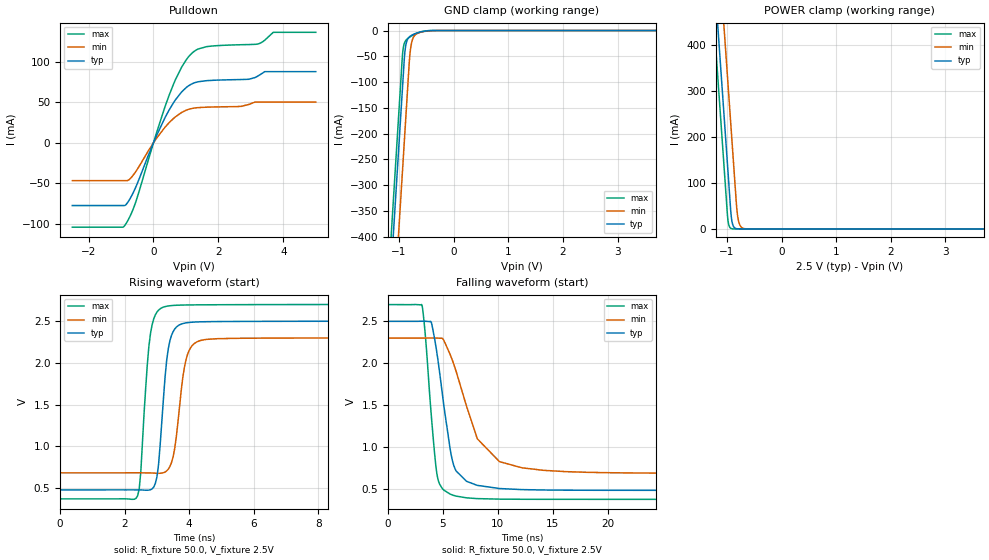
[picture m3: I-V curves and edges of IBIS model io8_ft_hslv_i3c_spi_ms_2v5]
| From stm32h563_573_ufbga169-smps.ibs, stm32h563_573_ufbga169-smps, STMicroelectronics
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[Model]   io8_ft_hslv_i3c_spi_ms_2v5
Model_type I/O_open_drain
Polarity   Non-Inverting
Enable   Active-Low
| CAP_THRESHOLD on pad IOFT is "UDTCAPC" :
| Rising=20.0% of vddiom   Falling=80.0% of vddiom
| C_comp min and max val. don't necessarily correlate with the min and max pvt
| but are the smallest and greatest pad capacitance found.
| var   typ   min   max
C_comp   3.87733pF  3.87281pF  3.96694pF
|C_comp_pulldown   3.87733pF  3.87281pF  3.96694pF
Vinl = 1.15V
Vinh = 1.35V
Vmeas = 1.25V   | Reference voltage for timing measurements
Cref  = 50.0pF   | Timing specification test load capacitance value
Rref  = 1.0MOhm   | Timing specification test load resistance value
Vref  = 1.375V   | Timing specification test load voltage
[Model Spec]
| TIME_THRESHOLD on pin ZII2CV11 is "CMOS" :
| Rising=40.0% of vdd   Falling=60.0% of vdd
Vinl 989.80000mV 917.80000mV 1.06580V
Vinh 1.40320V 1.29620V 1.49120V
| variable   typ   min   max
[Temperature Range] 25.0 125.0 -40.0
| variable   typ   min   max
[Voltage Range] 2.5V 2.3V 2.7V
| variable   typ   min   max
[POWER Clamp Reference] 2.5V 2.3V 2.7V
| variable   typ   min   max
[GND Clamp Reference] 0V 0V 0V
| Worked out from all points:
|   slope of the pulldown table from 0 to 0.375 V, typ, clamps not added: 11.5 ohm
|   GND clamp passes 1 mA (typ) near -0.52 V on its own axis
|   POWER clamp passes 1 mA (typ) near -0.84 V on its own axis
|   rising waveform, R_fixture 50.0, V_fixture 2.5V: 20-80 % time 254ps typ, 305ps min, 242ps max; typ from 0.481 V to 2.5 V
|   falling waveform, R_fixture 50.0, V_fixture 2.5V: 20-80 % time 1.3ns typ, 2.77ns min, 844ps max; typ from 2.5 V to 0.481 V
[POWER Clamp]
-2.5V     2.708A     2.899A     2.597A
-1.23V    548.8mA    740.2mA    437.5mA
-1.16V    429.8mA    621.2mA    318.5mA
-1.12V    361.8mA    553.2mA    250.5mA
-1.03V    208.8mA    400.2mA    97.53mA
-980mV    123.8mA    315.2mA    17.95mA
-920mV    26.3mA     213.2mA    906uA
-880mV    5.543mA    145.2mA    123.7uA
-810mV    363.5uA    33.6mA     3.797uA
-770mV    76.62uA    10.47mA    518.8nA
-700mV    5.026uA    1.361mA    16.11nA
5V        0A         0A         0A
[GND Clamp]
-2.5V     -2.77A     -2.931A    -2.704A
-1.21V    -576.8mA   -738.1mA   -511.3mA
-950mV    -134.8mA   -296.1mA   -69.34mA
-920mV    -83.82mA   -245.1mA   -32.48mA
-900mV    -50.56mA   -211.1mA   -24.02mA
-880mV    -31.31mA   -177.1mA   -19.85mA
-850mV    -18.7mA    -126.1mA   -16.34mA
-800mV    -11.46mA   -46.18mA   -12.45mA
-750mV    -8.203mA   -16.63mA   -9.325mA
-650mV    -4.063mA   -4.987mA   -4.427mA
-360mV    -35.05uA   -165.1uA   -9.564uA
5V        7.96nA     1.281uA    294pA
| variable   typ   min   max
[Pullup Reference] 2.5V 2.3V 2.7V
| variable   typ   min   max
[Pulldown Reference] 0V 0V 0V
[Pulldown]
-2.5V     -77.63mA   -46.85mA   -104.3mA
-870mV    -77.24mA   -46.85mA   -101.4mA
-550mV    -55.3mA    -35.88mA   -73.72mA
90mV      8.401mA    5.299mA    11.79mA
610mV     49.03mA    29.76mA    71.69mA
870mV     62.92mA    37.48mA    93.62mA
1.23V     73.63mA    42.72mA    112.2mA
1.64V     76.78mA    44.01mA    118.8mA
2.7V      78.15mA    44.99mA    121.2mA
3.22V     82.58mA    50.35mA    122.2mA
3.69V     87.93mA    50.35mA    136.5mA
5V        87.93mA    50.35mA    136.5mA
[Ramp]
dV/dt_r 1.21162V/249.69935ps 969.22666mV/302.34194ps 1.39626V/238.71411ps
dV/dt_f 1.21165V/1.30237ns 969.26055mV/2.47948ns 1.39628V/843.263ps
R_load = 50.0
| Removed startup time: 0s 0s 0s  .
| Removed end time: 34.4ns.
[Rising Waveform]
R_fixture   = 50.0
V_fixture   = 2.5V
V_fixture_min = 2.3V
V_fixture_max = 2.7V
0s        480.6mV    684.6mV    372.9mV
2.4ns     480.4mV    684.7mV    409.7mV
2.5ns     480mV      684.6mV    696.6mV
2.8ns     481.7mV    683.1mV    2.352V
3.05ns    783.7mV    678.8mV    2.632V
3.35ns    2.167V     727.8mV    2.682V
3.55ns    2.406V     973.3mV    2.69V
3.9ns     2.48V      2.037V     2.694V
4.5ns     2.494V     2.28V      2.696V
34.4ns    2.5V       2.3V       2.7V
| Removed startup time: 0s 0s 0s  .
| Removed end time: 99.4ns.
[Falling Waveform]
R_fixture   = 50.0
V_fixture   = 2.5V
V_fixture_min = 2.3V
V_fixture_max = 2.7V
0s        2.5V       2.3V       2.7V
3.1ns     2.501V     2.3V       2.69V
3.95ns    2.483V     2.301V     1.359V
4.5ns     2.079V     2.299V     640.9mV
5.65ns    979.4mV    2.106V     435.9mV
6.2ns     711.9mV    1.903V     411.6mV
8.15ns    539.3mV    1.094V     381.4mV
10.15ns   501.9mV    823.5mV    375.2mV
14.2ns    484.3mV    719mV      373.1mV
99.4ns    480.6mV    684.6mV    372.9mV
